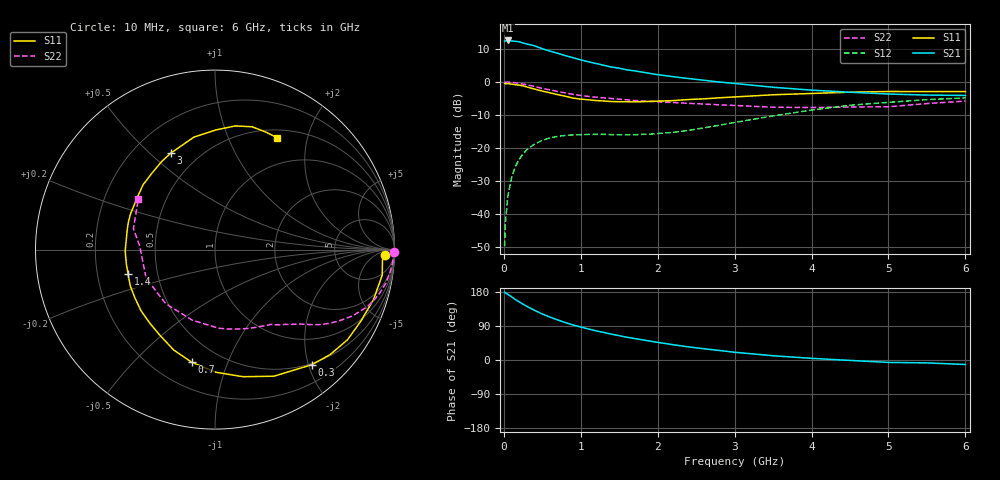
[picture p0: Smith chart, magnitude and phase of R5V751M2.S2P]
! SIEMENS Small Signal Semiconductors
! BFR183
! Si NPN RF Bipolar Junction Transistor in SOT23
! VCE = 0.75 V  IC = 1.2 mA
! Common Emitter S-Parameters:  May  1996
# GHz  S  MA  R  50
!  f  S11  S21  S12  S22
! GHz  MAG  ANG  MAG  ANG  MAG  ANG  MAG  ANG
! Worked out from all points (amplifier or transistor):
!   36 points, 10 MHz to 6 GHz, reference 50 ohm
!   highest |S21| = 12.6 dB at 50 MHz (marker M1)
!   |S21| within 3 dB of that: start of sweep to 566.3 MHz
!   unconditionally stable (mu >= 1): 1.544 GHz to 3.328 GHz
!   at 250 MHz: K = 0.17, MSG = 16.8 dB, |S12| = -21.9 dB
!   at 1.4 GHz: K = 0.92, MSG = 10.3 dB, |S12| = -16.0 dB
!   at 6 GHz: K = 0.99, MSG = 0.4 dB, |S12| = -4.8 dB
!   S11 on the Smith chart (normalised r, x): 10 MHz: 27, -15; 300 MHz: 0.48, -2.06; 700 MHz: 0.35, -0.75; 1.4 GHz: 0.34, -0.12; 3 GHz: 0.35, +0.58; 6 GHz: 0.60, +1.52
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0.01  0.9451 -1.8  4.158 179.1  0.0032 86.2  0.9967 -0.8
0.02  0.9349 -3.7  4.165 177.3  0.0071 89.0  0.9884 -1.4
0.05  0.9425 -8.7  4.261 173.4  0.0176 84.6  0.9937 -3.8
0.1  0.926 -17.5  4.184 167.0  0.0348 80.1  0.9825 -7.6
0.15  0.9054 -26.0  4.136 159.6  0.0518 74.6  0.9693 -11.3
0.2  0.8931 -34.2  4.066 153.4  0.0668 69.6  0.9503 -14.6
0.3  0.8381 -49.9  3.767 141.4  0.0936 61.1  0.9049 -20.7
0.4  0.7779 -65.1  3.531 131.1  0.1139 53.6  0.85 -25.8
0.5  0.725 -77.6  3.188 121.3  0.1293 47.3  0.797 -29.9
0.6  0.6834 -89.6  2.933 113.2  0.1412 42.2  0.7557 -33.0
0.7  0.6402 -101.8  2.719 105.7  0.149 38.1  0.7164 -35.7
0.9  0.5681 -122.5  2.329 92.4  0.1568 32.1  0.6467 -40.0
1.1  0.5348 -140.4  2.024 81.9  0.1594 28.7  0.6023 -43.7
1.4  0.5033 -164.3  1.681 68.1  0.1583 26.6  0.56 -48.5
1.7  0.4973 174.5  1.469 56.6  0.1576 30.0  0.5194 -53.3
2.2  0.5198 147.3  1.201 40.3  0.1714 37.9  0.4862 -63.5
3  0.591 114.7  0.948 20.4  0.242 45.5  0.4387 -87.3
3.5  0.6378 100.6  0.829 11.2  0.3045 43.2  0.413 -107.9
4.5  0.6982 80.7  0.697 -1.1  0.4417 30.6  0.4156 -157.6
5  0.7149 73.2  0.654 -6.4  0.4895 21.3  0.419 177.6
5.5  0.7134 66.4  0.631 -7.6  0.5374 15.5  0.4691 165.6
6  0.7131 61.1  0.623 -11.9  0.5731 6.3  0.5114 146.7
